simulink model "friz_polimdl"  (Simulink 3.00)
settings: Solver=ode45  StartTime=0.0  StopTime=10.0  RelTol=1e-5
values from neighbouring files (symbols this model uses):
  A = 1    [friz_poli.m]    (also in friz_acker.m)
  Kv = a    (= 1)    [friz_poli.m]    (also in friz_acker.m)
  P10 = 0    [friz_poli.m]    (also in friz_acker.m)
  Pm = 50    [friz_poli.m]
  x0 = 0    [friz_poli.m]    (also in friz_acker.m)
undefined symbols (not defined in the file or in its folder): b, Cm, Km, mp

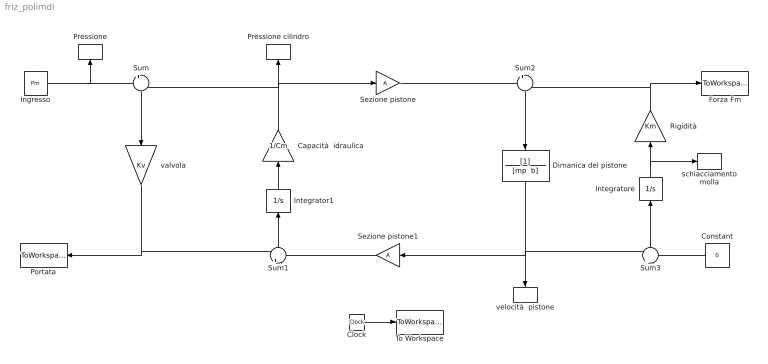
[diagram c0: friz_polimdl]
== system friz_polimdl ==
  Capacità  idraulica : Gain  Orientation=up  Gain=1/Cm  SaturateOnIntegerOverflow=on
  Clock : Clock
  Constant : Constant  Orientation=left  Value=0
  Dimanica del pistone : TransferFcn  Orientation=down  Numerator=[1]  Denominator="[mp  b]"
  Forza Fm : ToWorkspace  VariableName=Fm  SampleTime=-1  SaveFormat=Matrix
  Ingresso : Constant  Value=Pm
  Integrator1 : Integrator  Orientation=up  ExternalReset=none  InitialConditionSource=internal  InitialCondition=P10  LimitOutput=off  UpperSaturationLimit=inf  LowerSaturationLimit=-inf  ShowSaturationPort=off  ShowStatePort=off  AbsoluteTolerance=auto
  Integratore : Integrator  Orientation=up  ExternalReset=none  InitialConditionSource=internal  InitialCondition=x0  LimitOutput=off  UpperSaturationLimit=inf  LowerSaturationLimit=-inf  ShowSaturationPort=off  ShowStatePort=off  AbsoluteTolerance=auto
  Portata : ToWorkspace  VariableName=Q  SampleTime=-1  SaveFormat=Matrix
  Pressione : ToWorkspace  VariableName=P  SampleTime=-1  SaveFormat=Matrix
  Pressione cilindro : ToWorkspace  VariableName=P1  SampleTime=-1  SaveFormat=Matrix
  Rigidità : Gain  Orientation=up  Gain=Km  SaturateOnIntegerOverflow=on
  Sezione pistone : Gain  Gain=A  SaturateOnIntegerOverflow=on
  Sezione pistone1 : Gain  Orientation=left  Gain=A  SaturateOnIntegerOverflow=on
  Sum : Sum  Orientation=down  Inputs=+-  SaturateOnIntegerOverflow=on
  Sum1 : Sum  Orientation=up  Inputs=+-  SaturateOnIntegerOverflow=on
  Sum2 : Sum  Orientation=down  Inputs=+-  SaturateOnIntegerOverflow=on
  Sum3 : Sum  Orientation=up  Inputs=+-  SaturateOnIntegerOverflow=on
  To Workspace : ToWorkspace  VariableName=t  SampleTime=-1  SaveFormat=Matrix
  schiacciamento molla : ToWorkspace  VariableName=x  SampleTime=-1  SaveFormat=Matrix
  valvola : Gain  Orientation=down  Gain=Kv  SaturateOnIntegerOverflow=on
  velocità  pistone : ToWorkspace  VariableName=xdot  SampleTime=-1  SaveFormat=Matrix
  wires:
  Sum/1 -> valvola/1
  Sum1/1 -> Integrator1/1
  Integratore/1 -> Rigidità/1, schiacciamento molla/1
  Sum3/1 -> Integratore/1
  Sum2/1 -> Dimanica del pistone/1
  Sezione pistone/1 -> Sum2/1
  Sezione pistone1/1 -> Sum1/2
  Rigidità/1 -> Sum2/2, Forza Fm/1
  Dimanica del pistone/1 -> Sum3/1, Sezione pistone1/1, velocità  pistone/1
  Constant/1 -> Sum3/2
  Clock/1 -> To Workspace/1
  Capacità  idraulica/1 -> Sezione pistone/1, Sum/2, Pressione cilindro/1
  Integrator1/1 -> Capacità  idraulica/1
  Ingresso/1 -> Sum/1, Pressione/1
  valvola/1 -> Portata/1, Sum1/1
